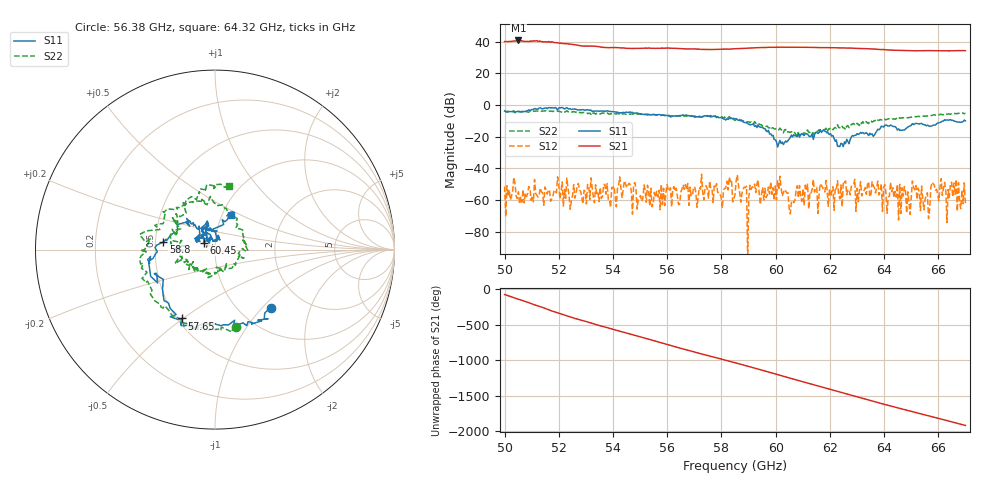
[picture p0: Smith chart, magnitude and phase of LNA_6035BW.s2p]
!Agilent Technologies,E8361A,US42410132,A.06.03.05
!Agilent E8361A: A.06.03.05
!Date: Friday, July 11, 2008 12:53:24
!Correction: S11(Full 2 Port(1,2)) S21(Full 2 Port(1,2)) S12(Full 2 Port(1,2)) S22(Full 2 Port(1,2))
!S2P File: Measurements: S11, S21, S12, S22:
# Hz S  MA  R 50
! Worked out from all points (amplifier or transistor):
!   401 points, 50 GHz to 67 GHz, reference 50 ohm
!   highest |S21| = 40.8 dB at 50.51 GHz (marker M1)
!   |S21| within 3 dB of that: start of sweep to 52.69 GHz
!   unconditionally stable (mu >= 1): 52.58 GHz to 53.05 GHz; 53.23 GHz to 54.42 GHz; 54.43 GHz to end of sweep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
!   at 52.8 GHz: K = 1.54, MAG = 41.6 dB, |S12| = -54.5 dB
!   at 58.5 GHz: K = 4.54, MAG = 36.5 dB, |S12| = -56.6 dB
!   at 67 GHz: K = 7.71, MAG = 36.3 dB, |S12| = -62.1 dB
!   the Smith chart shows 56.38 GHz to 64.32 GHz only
!   S11 on the Smith chart (normalised r, x): 56.38 GHz: 1.38, -1.13; 57.65 GHz: 0.53, -0.49; 58.8 GHz: 0.55, +0.05; 60.45 GHz: 0.88, +0.07; 64.32 GHz: 1.10, +0.44
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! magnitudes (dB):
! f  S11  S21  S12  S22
! 50 GHz  -3.8  40.0  -51.5  -3.6
! 50.51 GHz  -4.0  40.8  -54.9  -4.1
! 52.04 GHz  -1.8  39.0  -59.4  -4.1
! 52.85 GHz  -3.0  37.2  -58.6  -4.9
! 54.51 GHz  -4.6  35.8  -52.3  -5.9
! 54.97 GHz  -5.5  35.8  -58.5  -5.8
! 55.7 GHz  -6.1  35.8  -53.9  -6.3
! 56.38 GHz  -6.9  35.7  -57.8  -6.9
! 57.65 GHz  -7.4  35.0  -52.9  -7.6
! 58.5 GHz  -8.8  35.5  -56.6  -9.8
! 58.8 GHz  -10.7  35.8  -53.4  -9.9
! 60.16 GHz  -22.4  36.5  -45.1  -14.7
! 60.45 GHz  -22.5  36.5  -55.5  -17.0
! 61.35 GHz  -18.2  36.3  -53.3  -16.9
! 62.41 GHz  -24.2  36.1  -50.5  -14.9
! 64.19 GHz  -13.4  34.7  -57.7  -8.7
! 64.32 GHz  -13.5  34.7  -52.4  -8.8
! 64.92 GHz  -13.5  34.4  -61.0  -8.0
! 65.09 GHz  -12.4  34.2  -51.9  -7.6
! 65.6 GHz  -12.8  34.3  -55.5  -6.9
! 65.81 GHz  -12.8  34.3  -49.8  -6.4
! 67 GHz  -10.0  34.3  -62.1  -5.2
